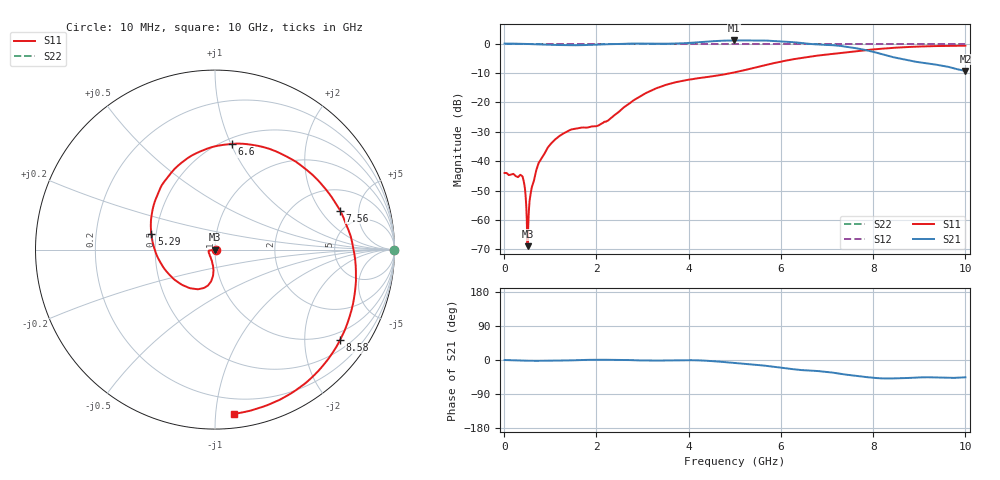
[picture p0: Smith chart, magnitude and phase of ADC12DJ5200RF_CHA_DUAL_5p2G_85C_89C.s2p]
! Texas Instruments, Inc.
! ADC12DJ5200RF - CH A S-Parameters (Dual Ch Mode, Fs = 5.2 GSPS, 85 degC case, 89 degC juntion)
! Port 1 represents the 100-ohm differenal input, Port 2 the digital output
! freq  dbS11  angS11  dbS21 angS21 dbS12 angS12 dbS22 angS22
# HZ S DB R 100
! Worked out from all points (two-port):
!   1000 points, 10 MHz to 10 GHz, reference 100 ohm
!   highest |S21| = 1.06 dB at 4.99 GHz (marker M1); lowest = -9.3 dB at 10 GHz (marker M2)
!   |S21| within 3 dB of the highest: start of sweep to 7.756 GHz
!   lowest |S11| = -68.9 dB at 510 MHz (marker M3), VSWR 1.00, Z = 100 - j0.0713 ohm
!   |S11| at or under -10 dB: start of sweep to 4.932 GHz
!   |S22| runs from 0.0 to 0.0 dB; largest |S21 - S12| = 0.8
!   S11 on the Smith chart (normalised r, x): 10 MHz: 1.01, -0.00; 5.29 GHz: 0.47, +0.10; 6.6 GHz: 0.55, +1.01; 7.56 GHz: 3.35, +3.13; 8.58 GHz: 0.75, -2.91; 10 GHz: 0.09, -1.12
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1e7  -43.98 -7.6  0.00 -0.0  0.00 0.0  0.00 0.0
3.8e8  -44.92 -10.5  -0.07 -1.6  0.00 0.0  0.00 0.0
4.3e8  -47.24 -0.5  -0.10 -1.8  0.00 0.0  0.00 0.0
4.7e8  -52.81 6.8  -0.12 -1.9  0.00 0.0  0.00 0.0
5.1e8  -68.87 -81.6  -0.14 -2.0  0.00 0.0  0.00 0.0
7.1e8  -42.37 -157.4  -0.26 -2.1  0.00 0.0  0.00 0.0
9.4e8  -35.52 -169.1  -0.36 -2.1  0.00 0.0  0.00 0.0
1.26e9  -30.80 -171.7  -0.51 -1.5  0.00 0.0  0.00 0.0
1.68e9  -28.56 -163.4  -0.53 0.0  0.00 0.0  0.00 0.0
2.24e9  -26.25 -119.8  -0.22 0.4  0.00 0.0  0.00 0.0
3.34e9  -14.98 -96.9  -0.03 -1.5  0.00 0.0  0.00 0.0
4.23e9  -11.74 -125.4  0.48 -1.0  0.00 0.0  0.00 0.0
4.99e9  -9.80 -173.0  1.06 -7.8  0.00 0.0  0.00 0.0
5.01e9  -9.74 -174.4  1.06 -8.0  0.00 0.0  0.00 0.0
5.29e9  -8.74 165.9  1.04 -10.7  0.00 0.0  0.00 0.0
5.9e9  -6.49 126.2  0.86 -18.8  0.00 0.0  0.00 0.0
6.6e9  -4.49 81.1  -0.04 -27.8  0.00 0.0  0.00 0.0
6.67e9  -4.33 76.5  -0.16 -28.4  0.00 0.0  0.00 0.0
7.56e9  -2.73 17.4  -1.40 -40.7  0.00 0.0  0.00 0.0
8.34e9  -1.56 -25.8  -4.24 -48.8  0.00 0.0  0.00 0.0
8.58e9  -1.31 -35.9  -5.08 -47.9  0.00 0.0  0.00 0.0
1e10  -0.71 -83.2  -9.31 -45.7  0.00 0.0  0.00 0.0
